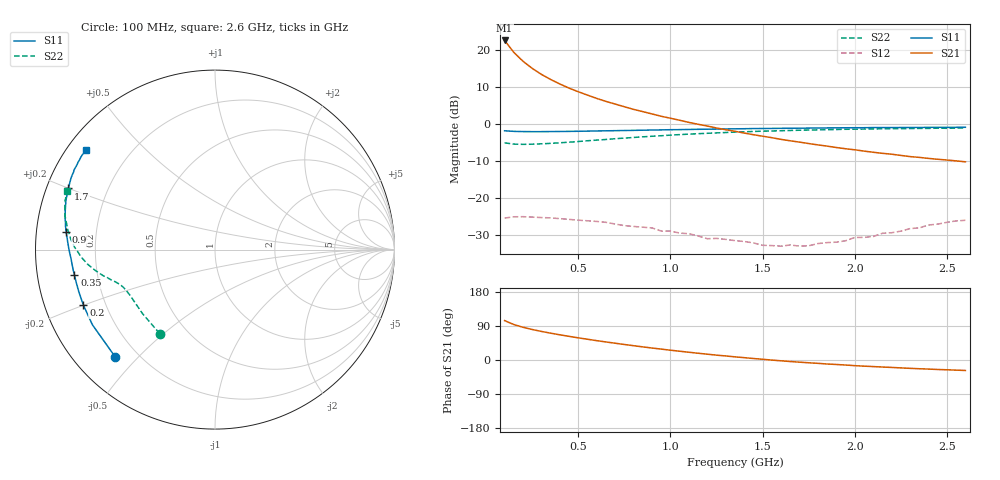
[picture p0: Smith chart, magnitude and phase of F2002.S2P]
!  POLYFET RF DEVICES
!  S PARAMETERS FOR
!  F2002
!  VDS=28, IDQ=400mA
! Date: Mon Aug  5 14:04:45 1991
# MHZ S MA R 50
! Bias (V mA) : V1=3.5470000  I1=0.0136700  V2=28.001700  I2=404.81880
!  FREQ  S11  S11 ANG  S21  S21 ANG  S12  S12 ANG  S22  S22 ANG
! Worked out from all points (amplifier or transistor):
!   51 points, 100 MHz to 2.6 GHz, reference 50 ohm
!   highest |S21| = 22.7 dB at 100 MHz (marker M1)
!   |S21| within 3 dB of that: start of sweep to 146.5 MHz
!   unconditionally stable (mu >= 1): 926.3 MHz to 2.449 GHz; 2.453 GHz to 2.509 GHz
!   at 500 MHz: K = 0.48, MSG = 17.4 dB, |S12| = -26.0 dB
!   at 1.35 GHz: K = 1.58, MAG = 10.3 dB, |S12| = -31.5 dB
!   at 2.6 GHz: K = 0.93, MSG = 7.9 dB, |S12| = -26.0 dB
!   S11 on the Smith chart (normalised r, x): 100 MHz: 0.12, -0.43; 200 MHz: 0.12, -0.20; 350 MHz: 0.11, -0.09; 900 MHz: 0.09, +0.06; 1.7 GHz: 0.06, +0.20; 2.6 GHz: 0.05, +0.34
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100  0.8163 -132.9  13.61 103.9  0.05378 18.4  0.5608 -123.2
150  0.8013 -148.5  9.385 93.5  0.05602 9.4  0.5387 -138.7
200  0.7959 -157.1  7.108 86.3  0.05618 3.3  0.5348 -146.9
250  0.7943 -162.7  5.694 80.5  0.05548 -0.9  0.5376 -151.8
300  0.7945 -166.8  4.724 75.4  0.05468 -3.2  0.5441 -155.2
350  0.7961 -169.8  4.033 70.8  0.05414 -6.0  0.5514 -157.5
400  0.7987 -172.3  3.502 66.4  0.05283 -8.3  0.5614 -159.5
450  0.801 -174.4  3.081 62.4  0.05162 -10.6  0.5721 -160.8
500  0.8035 -176.3  2.75 58.4  0.05036 -12.7  0.584 -162.2
550  0.8074 -177.9  2.478 54.7  0.04944 -15.5  0.598 -163.3
600  0.8118 -179.4  2.235 51.0  0.04841 -16.0  0.6105 -164.5
700  0.8191 177.9  1.875 44.3  0.04463 -18.0  0.6375 -166.7
800  0.8264 175.5  1.59 37.7  0.04143 -19.9  0.6625 -168.9
900  0.8355 173.2  1.379 31.6  0.03959 -20.3  0.6882 -171.1
950  0.839 172.1  1.282 28.7  0.0359 -21.3  0.6991 -172.2
1150  0.8545 167.8  0.999 17.8  0.03083 -16.4  0.7451 -176.7
1350  0.8676 163.8  0.8031 8.3  0.02663 -13.7  0.7834 178.9
1500  0.8761 160.9  0.689 1.9  0.02304 -4.8  0.8062 175.8
1700  0.8847 157.3  0.5732 -5.7  0.02245 13.2  0.8301 172.0
1800  0.8897 155.6  0.5257 -8.8  0.02432 21.0  0.8391 170.1
2200  0.9019 148.9  0.3934 -19.6  0.03406 38.3  0.8712 163.7
2600  0.9102 142.2  0.3104 -27.6  0.05021 42.2  0.8897 158.4
